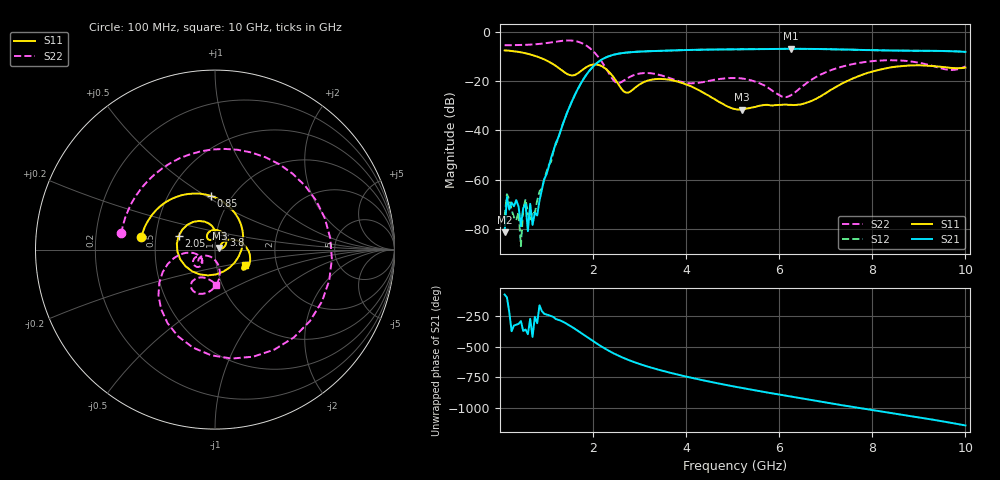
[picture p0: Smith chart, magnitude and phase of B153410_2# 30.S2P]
!  2-Port S-parameters saved by WinCal
! VAR MeasName=S-Parameters (CALIBRATED_DATA) read from VNA (N5245A)
! VAR MeasDate=2016-12-23 10:00:53
! VAR NAME=B153410_2# 30
! VAR FILENAME=B153410_2# 30.S2P
! VAR DATE=2016-12-23 10:00:53
! VAR PHYS_PORTS=1,2
# Hz S DB R 50
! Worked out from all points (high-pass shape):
!   199 points, 100 MHz to 10 GHz, reference 50 ohm
!   highest |S21| = -6.96 dB at 6.25 GHz (marker M1); lowest = -81.3 dB at 100 MHz (marker M2)
!   |S21| within 3 dB of the highest: 2.341 GHz to end of sweep
!   lowest |S11| = -31.6 dB at 5.2 GHz (marker M3), VSWR 1.05, Z = 52.5 + j1.01 ohm
!   |S11| at or under -10 dB: 780.2 MHz to end of sweep
!   |S22| runs from -26.6 to -3.6 dB; largest |S21 - S12| = 0.0041
!   S11 on the Smith chart (normalised r, x): 100 MHz: 0.42, +0.07; 850 MHz: 0.80, +0.53; 2.05 GHz: 0.66, +0.10; 3.8 GHz: 1.09, +0.18; 10 GHz: 1.37, -0.25
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1e8  -7.62 170.4  -81.31 -77.5  -75.19 64.9  -5.51 170.2
1.5e8  -7.68 165.6  -67.07 -100.8  -65.90 96.0  -5.51 165.3
3.5e8  -8.06 146.2  -68.32 37.1  -76.55 -48.0  -5.47 145.0
4e8  -8.21 141.3  -70.91 44.0  -73.17 -38.7  -5.44 139.8
4.5e8  -8.37 136.4  -78.91 67.1  -86.99 106.8  -5.42 134.4
5.5e8  -8.77 126.4  -70.03 -1.8  -67.97 -26.4  -5.36 123.1
6e8  -8.99 121.2  -80.90 -39.5  -73.71 117.4  -5.31 117.2
6.5e8  -9.25 116.1  -69.83 85.6  -76.90 -28.4  -5.26 111.2
7e8  -9.52 110.9  -78.37 -61.3  -72.87 153.6  -5.21 104.8
8.5e8  -10.47 94.1  -68.46 -164.8  -64.81 -179.0  -4.98 84.4
1.35e9  -15.96 12.6  -37.57 62.4  -37.49 61.7  -3.70 -4.4
1.75e9  -15.82 -121.3  -20.63 -30.8  -20.60 -30.6  -4.59 -92.1
2.05e9  -13.30 159.5  -13.27 -107.6  -13.26 -107.7  -8.86 -149.3
2.5e9  -20.07 89.9  -9.10 154.3  -9.11 154.3  -20.73 -155.0
3.4e9  -19.18 92.4  -7.81 32.9  -7.81 32.9  -17.43 -153.8
3.8e9  -20.17 58.6  -7.56 -5.9  -7.57 -5.8  -19.81 -157.6
5.05e9  -31.41 15.5  -7.17 -105.6  -7.18 -105.4  -18.81 -143.3
5.2e9  -31.58 21.4  -7.14 -116.1  -7.15 -116.0  -18.99 -146.4
6.25e9  -29.69 21.9  -6.96 173.7  -6.98 173.7  -25.81 -101.0
6.7e9  -28.07 36.8  -6.99 144.6  -7.02 144.6  -19.45 -77.1
8.35e9  -14.65 -1.3  -7.64 44.0  -7.65 44.4  -11.59 -112.3
1e10  -14.56 -28.3  -8.20 -60.4  -8.22 -60.0  -14.11 -88.2
